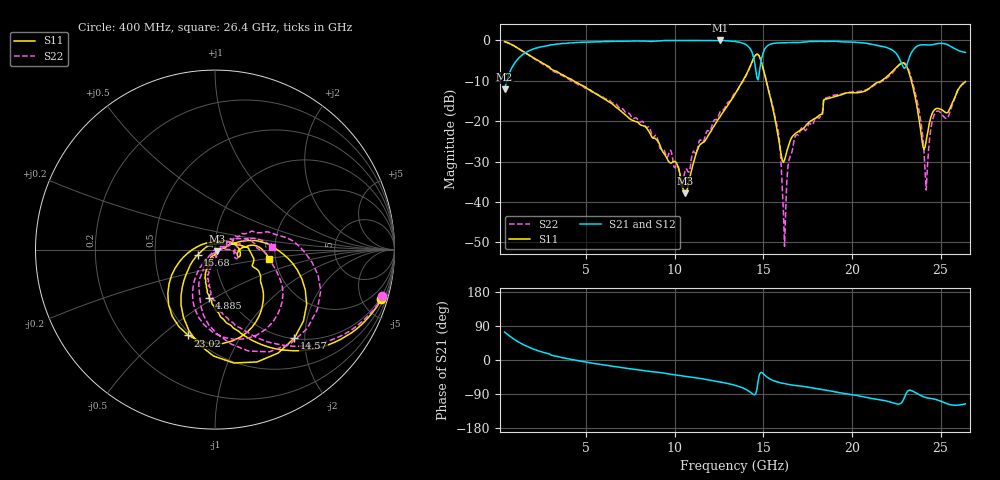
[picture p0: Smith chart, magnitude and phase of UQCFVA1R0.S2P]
!  Part Number  UQCFVA1R0  Mounting Orientation: Horizontal
!  Description: Ultra Low ESR Microwave capacitors
!  Application: Coupling, Bypass, Tuning, DC Block
!  Filters, Matching
# GHZ S DB R 50
! Freq  |S11|  S11 Ph  |S21|  S21 Ph  |S12|  S12 Ph  |S22|  S22 Ph
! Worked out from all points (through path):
!   401 points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, 400 MHz to 26.4 GHz, reference 50 ohm
!   highest |S21| = 0.00 dB at 12.55 GHz (marker M1); lowest = -12.1 dB at 400 MHz (marker M2)
!   group delay of S21, straight-line fit = 16.3 ps
!   lowest |S11| = -37.9 dB at 10.61 GHz (marker M3), VSWR 1.03, Z = 51 - j0.87 ohm
!   |S11| at or under -10 dB: 4.282 GHz to 13.84 GHz (9.554 GHz wide, 105 % of centre); 15.16 GHz to 21.66 GHz (6.501 GHz wide, 35.3 % of centre); 23.35 GHz to end of sweep
!   |S22| runs from -51.0 to -0.3 dB; largest |S21 - S12| = 0.003
!   S11 on the Smith chart (normalised r, x): 400 MHz: 0.78, -6.72; 4.885 GHz: 0.81, -0.47; 14.57 GHz: 1.01, -1.78; 15.68 GHz: 0.82, -0.05; 23.02 GHz: 0.48, -0.62; 26.4 GHz: 1.85, -0.22
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0.4  -0.29 -16.7  -12.11 73.7  -12.09 73.6  -0.28 -15.6
2.285  -4.97 -66.1  -1.76 24.5  -1.75 24.5  -5.14 -63.6
4.755  -11.13 -95.6  -0.44 -3.7  -0.43 -3.7  -11.17 -92.6
4.885  -11.35 -96.9  -0.41 -4.6  -0.40 -4.6  -11.64 -93.3
9.11  -25.38 -118.2  -0.13 -32.8  -0.13 -32.9  -25.88 -101.0
10.605  -37.87 -41.9  -0.01 -43.1  -0.01 -43.1  -31.87 -13.8
12.555  -18.90 18.6  0.00 -57.8  -0.01 -57.8  -17.73 30.9
13.4  -13.32 13.6  -0.26 -66.7  -0.26 -66.7  -12.89 26.8
14.18  -7.16 -10.0  -1.62 -82.2  -1.62 -82.2  -7.21 6.5
14.57  -3.58 -48.1  -7.23 -89.1  -7.24 -89.0  -3.60 -30.3
15.025  -7.62 -115.0  -2.62 -37.6  -2.63 -37.6  -7.52 -94.8
15.675  -19.83 -162.8  -0.67 -56.3  -0.67 -56.2  -19.31 -124.5
16.195  -29.58 74.3  -0.56 -62.4  -0.57 -62.4  -50.96 -122.3
16.78  -23.18 20.2  -0.53 -67.1  -0.53 -67.1  -23.93 21.2
17.755  -19.75 17.8  -0.25 -73.8  -0.25 -73.7  -20.95 26.7
18.535  -14.49 1.2  -0.24 -79.5  -0.25 -79.4  -14.25 17.5
22.11  -8.39 -44.9  -2.00 -110.3  -2.01 -110.2  -8.79 -19.4
23.02  -6.01 -107.3  -6.71 -91.8  -6.72 -91.7  -5.81 -77.6
23.67  -16.41 -173.1  -1.45 -88.5  -1.46 -88.5  -14.81 -125.7
24.19  -24.79 57.0  -1.09 -99.3  -1.10 -99.2  -37.03 -57.9
24.645  -17.25 -1.9  -0.94 -103.1  -0.94 -103.0  -18.37 -9.8
26.4  -10.25 -10.0  -2.95 -115.6  -2.95 -115.4  -9.90 2.8
